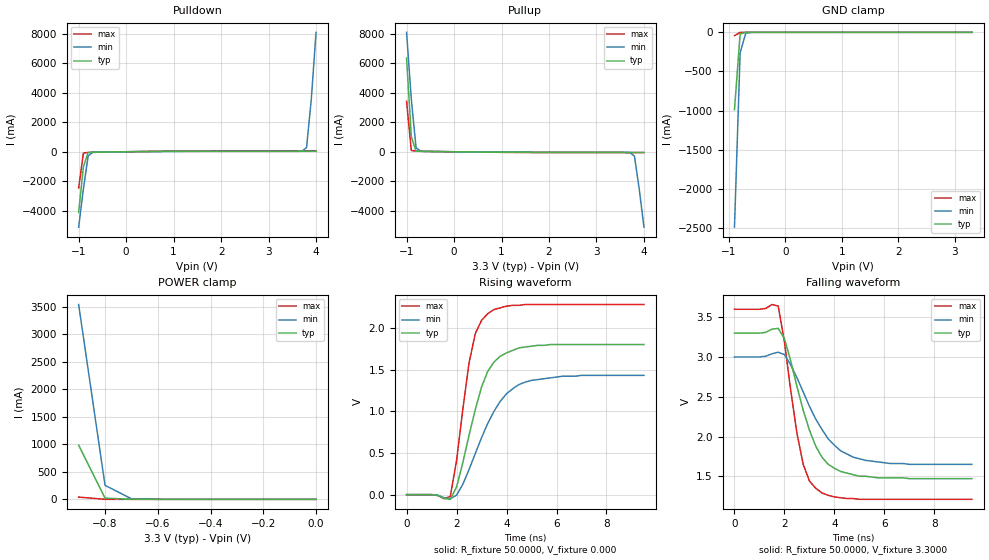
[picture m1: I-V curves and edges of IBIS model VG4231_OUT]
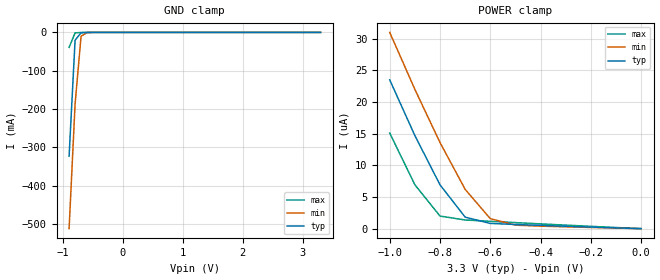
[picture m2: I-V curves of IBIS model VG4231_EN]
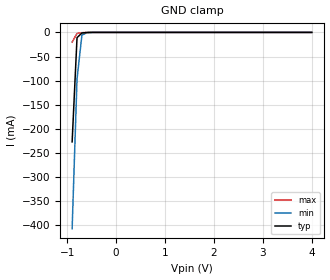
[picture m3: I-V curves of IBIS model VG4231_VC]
[IBIS ver]   2.1
[File name]   423acacz.ibs
[File Rev]   0.1
[Date]   November 12, 2007
[Copyright]   EPSONTOYOCOM Corp.
|   Component VG-4231CAxxC
[Component]   VG-4231CAxxC
[Manufacturer]   EPSONTOYOCOM Corp.
[Package]
| variable   typ   min   max
R_pkg   0.20   0.13   0.28
L_pkg   5.16nH   4.56nH   5.76nH
C_pkg   1.23pF   1.03pF   1.53pF
[Pin]  signal_name   model_name   R_pin   L_pin   C_pin
1   VC   VG4231_VC
2   OE   VG4231_EN
3   GND   GND
4   OUT   VG4231_OUT
5   NC   NC
6   VDD   POWER
| Models and submodels in the file (3): VG4231_OUT (3-state), VG4231_EN (Input), VG4231_VC (Input)
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|   Model VG4231_OUT
[Model]   VG4231_OUT
Model_type   3-state
Polarity   Non-Inverting
Enable   Active-High
C_comp   2.2010pF   2.2010pF   2.2010pF
[Temperature Range]   27.0000   85.0000   -40.0000
[Voltage Range]   3.3000V   3.0000V   3.6000V
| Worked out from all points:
|   slope of the pulldown table from 0 to 0.495 V, typ, clamps not added: 28.4 ohm
|   slope of the pullup table from 0 to 0.495 V, typ, clamps not added: 30.8 ohm
|   GND clamp passes 1 mA (typ) near -0.70 V on its own axis
|   POWER clamp passes 1 mA (typ) near -0.70 V on its own axis
|   rising waveform, R_fixture 50.0000, V_fixture 0.000: 20-80 % time 966ps typ, 1.34ns min, 655ps max; typ from 0 V to 1.8 V
|   falling waveform, R_fixture 50.0000, V_fixture 3.3000: 20-80 % time 1.07ns typ, 1.39ns min, 698ps max; typ from 3.3 V to 1.47 V
[Pulldown]
| voltage   I(typ)   I(min)   I(max)
-1V       -4.12A     -5.12A     -2.46A
-900mV    -1.02A     -2.52A     -91.6mA
-800mV    -54.2mA    -285mA     -45.6mA
-700mV    -29.3mA    -32.1mA    -39.8mA
1.2V      33.1mA     23.8mA     47.8mA
3.6V      41.7mA     30.2mA     59.7mA
3.7V      41.8mA     40.3mA     59.8mA
3.8V      41.8mA     284mA      59.8mA
3.9V      41.9mA     3.57A      59.9mA
4V        42.7mA     8.11A      59.9mA
[Pullup]
| voltage   I(typ)   I(min)   I(max)
-1V       6.36A      8.11A      3.43A
-900mV    1.02A      3.57A      86.9mA
-800mV    52.7mA     279mA      41.9mA
-700mV    28.1mA     32.6mA     36.2mA
-600mV    23.5mA     19.5mA     30.9mA
3.7V      -45.7mA    -45.3mA    -62.8mA
3.8V      -45.8mA    -295mA     -62.9mA
3.9V      -46.1mA    -2.53A     -63.1mA
4V        -47mA      -5.12A     -63.2mA
[GND_clamp]
| voltage   I(typ)   I(min)   I(max)
-900mV    -988mA     -2.49A     -42.8mA
-800mV    -22.3mA    -261mA     -1.3mA
-700mV    -968uA     -10.8mA    -315uA
-500mV    -14.7uA    -62uA      -1.68uA
3.3V      74.5pA     1.55uA     62.4pA
[POWER_clamp]
| voltage   I(typ)   I(min)   I(max)
--1.00 	6.32E+00	8.08E+00	3.38E+00
-900mV    985mA      3.54A      40.6mA
-800mV    21.5mA     254mA      540uA
-700mV    770uA      10.7mA     43.6uA
-600mV    84.6uA     712uA      4.3uA
-500mV    10.8uA     95.8uA     259nA
-400mV    1.01uA     13.7uA     7.7nA
-300mV    59.3nA     1.55uA     241pA
-200mV    2.49nA     124nA      92.5pA
-100mV    153pA      7.18nA     84.8pA
0V        74.5pA     170pA      79.2pA
[Ramp]
| variable   typ   min   max
dV/dt_r   1.08/0.963n   0.859/1.33n   1.37/0.635n
dV/dt_f   1.10/1.05n   0.812/1.40n   1.43/0.698n
R_load = 50.0000
[Rising Waveform]
R_fixture = 50.0000
V_fixture = 0.000
V_fixture_min = 0.000
V_fixture_max = 0.000
| time   V(typ)   V(min)   V(max)
0s        1.92nV     12.4nV     1.59nV
1.75ns    -56.3mV    -49.5mV    -22.8mV
2ns       90.8mV     -6.35mV    408mV
2.5ns     712mV      301mV      1.58V
2.75ns    1.02V      493mV      1.93V
3.25ns    1.48V      855mV      2.17V
4ns       1.7V       1.21V      2.26V
4.75ns    1.77V      1.35V      2.28V
6.25ns    1.8V       1.42V      2.28V
9.5ns     1.8V       1.43V      2.28V
[Falling Waveform]
R_fixture = 50.0000
V_fixture = 3.3000
V_fixture_min = 3.0000
V_fixture_max = 3.6000
| time   V(typ)   V(min)   V(max)
0s        3.3V       3V         3.6V
1.75ns    3.36V      3.06V      3.64V
2ns       3.23V      3.03V      3.19V
2.5ns     2.63V      2.74V      2.04V
2.75ns    2.33V      2.56V      1.65V
3ns       2.08V      2.38V      1.44V
3.25ns    1.88V      2.22V      1.35V
3.75ns    1.65V      1.97V      1.26V
4.75ns    1.52V      1.74V      1.22V
9.5ns     1.47V      1.65V      1.21V
|   Model VG4231_EN
[Model]   VG4231_EN
Model_type   Input
Vinl =   0.6600V
Vinh =   2.6400V
C_comp   1.4070pF   1.4070pF   1.4070pF
[Temperature Range]   27.0000   85.0000   -40.0000
[Voltage Range]   3.3000V   3.0000V   3.6000V
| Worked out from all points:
|   GND clamp passes 1 mA (typ) near -0.70 V on its own axis
[GND_clamp]
| voltage   I(typ)   I(min)   I(max)
-900mV    -323mA     -512mA     -39mA
-800mV    -20.3mA    -187mA     -1.24mA
-700mV    -916uA     -9.88mA    -313uA
-600mV    -139uA     -599uA     -39.6uA
-500mV    -16.2uA    -62uA      -3.84uA
3.3V      18.4pA     290nA      -498nA
[POWER_clamp]
| voltage   I(typ)   I(min)   I(max)
-1V       23.5uA     31uA       15.1uA
-900mV    14.7uA     22uA       6.93uA
-800mV    6.92uA     13.6uA     1.99uA
-700mV    1.82uA     6.21uA     1.37uA
-600mV    828nA      1.58uA     1.16uA
-500mV    659nA      555nA      954nA
-400mV    518nA      396nA      753nA
-300mV    382nA      290nA      557nA
-200mV    250nA      189nA      366nA
-100mV    123nA      92.7nA     180nA
0V        18.4pA     119pA      18pA
|   Model VG4231_VC
[Model]   VG4231_VC
Model_type   Input
Vinl =   0.800V
Vinh =   2.000V
C_comp   1.4070pF   1.4070pF   1.4070pF
[Temperature Range]   27.0000   85.0000   -40.0000
[Voltage Range]   3.3000V   3.0000V   3.6000V
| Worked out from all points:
|   GND clamp passes 1 mA (typ) near -0.67 V on its own axis
[GND_clamp]
| voltage   I(typ)   I(min)   I(max)
-900mV    -227mA     -407mA     -20.1mA
-800mV    -11mA      -96.7mA    -2.11mA
-700mV    -1.25mA    -5.64mA    -622uA
-600mV    -265uA     -674uA     -75.4uA
-500mV    -29.8uA    -103uA     -3.49uA
4V        12.3pA     250pA      8pA
